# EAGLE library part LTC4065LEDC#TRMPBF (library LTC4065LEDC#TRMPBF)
Battery Management Standalone 250mA Li-Ion Coin Cell Charger Source: Datasheet
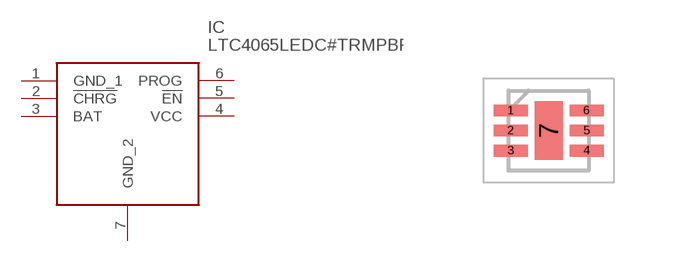
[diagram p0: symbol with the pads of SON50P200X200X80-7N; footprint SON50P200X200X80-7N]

Designator prefix IC

## LTC4065LEDC#TRMPBF (Description: Battery Management Standalone 250mA Li-Ion Coin Cell Charger; Height: 0.8mm; Manufacturer_Name: Analog Devices; Manufacturer_Part_Number: LTC4065LEDC#TRMPBF; Mouser_Part_Number: 584-C4065LEDCTRMPBF; Mouser_Price-Stock: https://www.mouser.co.uk/ProductDetail/Analog-Devices/LTC4065LEDCTRMPBF?qs=hVkxg5c3xu8%2FWtpri9P%2FRQ%3D%3D)  [SON50P200X200X80-7N]
1  GND_1
2  !CHRG
3  BAT
4  VCC
5  !EN
6  PROG
7  GND_2

## Footprint SON50P200X200X80-7N (pad centres in mm)
DC6 Package
smd 0.85 x 0.3: 1 -0.95,0.5; 2 -0.95,0; 3 -0.95,-0.5; 4 0.95,-0.5; 5 0.95,0; 6 0.95,0.5
smd 0.7 x 1.47: 7 0,0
